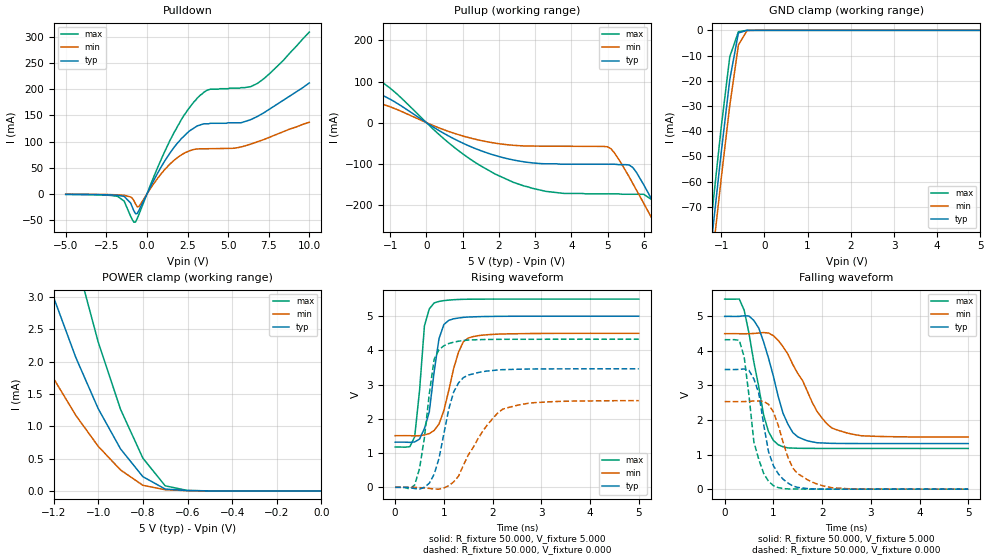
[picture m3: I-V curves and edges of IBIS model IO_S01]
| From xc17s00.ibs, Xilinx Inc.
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|   Model IO_S01
[Model]   IO_S01
Model_type   I/O
Polarity   Non-Inverting
Enable   Active-High
Vinl =   0.800V
Vinh =   2.000V
Vmeas =   2.500V
Cref =  50.000pF
Rref =   1.000M
Vref =  0.000V
C_comp   2.750pF   2.250pF   3.250pF
[Temperature Range]   50.000   100.000   0.000
[Voltage Range]   5.000V   4.500V   5.500V
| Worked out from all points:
|   slope of the pulldown table from 0 to 0.75 V, typ, clamps not added: 16.8 ohm
|   slope of the pullup table from 0 to 0.75 V, typ, clamps not added: 19.3 ohm
|   GND clamp passes 1 mA (typ) near -0.59 V on its own axis
|   POWER clamp passes 1 mA (typ) near -0.96 V on its own axis
|   rising waveform, R_fixture 50.000, V_fixture 5.000: 20-80 % time 222ps typ, 325ps min, 154ps max; typ from 1.32 V to 5 V
|   rising waveform, R_fixture 50.000, V_fixture 0.000: 20-80 % time 331ps typ, 657ps min, 237ps max; typ from 0 V to 3.46 V
|   falling waveform, R_fixture 50.000, V_fixture 5.000: 20-80 % time 444ps typ, 672ps min, 339ps max; typ from 5 V to 1.32 V
|   falling waveform, R_fixture 50.000, V_fixture 0.000: 20-80 % time 296ps typ, 409ps min, 267ps max; typ from 3.46 V to 0 V
[Pulldown]
| voltage   I(typ)   I(min)   I(max)
-5V       -500uA     -400uA     -700uA
-1.8V     -2.5mA     -1.6mA     -4.5mA
-1.4V     -4.5mA     -2.4mA     -13.5mA
-1V       -17.19mA   -5.5mA     -42.5mA
-700mV    -37.46mA   -18.93mA   -53.28mA
-500mV    -31.8mA    -24.06mA   -39.58mA
1.4V      77.3mA     56.57mA    101mA
3.1V      130mA      86.12mA    183mA
3.9V      135mA      86.54mA    200mA
5.8V      136mA      89.89mA    203mA
6.8V      148mA      99.73mA    211mA
10V       212mA      137mA      309mA
[Pullup]
| voltage   I(typ)   I(min)   I(max)
-5V       138mA      75.48mA    233mA
-3.8V     136mA      79.24mA    211mA
-2.2V     104mA      68.39mA    154mA
-1V       56.81mA    38.43mA    83.6mA
1V        -49.62mA   -32.24mA   -75.63mA
2.4V      -90.7mA    -55.01mA   -145mA
3.3V      -100mA     -57.13mA   -167mA
5V        -101mA     -58.64mA   -173mA
5.7V      -109mA     -148mA     -174mA
6.4V      -215mA     -261mA     -198mA
6.8V      -281mA     -327mA     -262mA
10V       -833mA     -863mA     -828mA
[GND_clamp]
| voltage   I(typ)   I(min)   I(max)
-5V       -728mA     -719mA     -739mA
-1.4V     -113mA     -121mA     -104mA
-1.2V     -80.19mA   -89.89mA   -70.7mA
-1V       -48.75mA   -59.03mA   -38.71mA
-800mV    -19.55mA   -29.76mA   -10.47mA
-600mV    -1.037mA   -5.805mA   -545uA
-400mV    -3.699uA   -72.4uA    -2.038uA
5V        350pA      999nA      143pA
[POWER_clamp]
| voltage   I(typ)   I(min)   I(max)
-5V       71.66mA    42.52mA    116mA
-1.4V     5.246mA    3.126mA    8.7mA
-1.3V     4.067mA    2.398mA    6.818mA
-1.2V     3.001mA    1.742mA    5.11mA
-1.1V     2.064mA    1.169mA    3.598mA
-1V       1.274mA    691uA      2.306mA
-900mV    651uA      325uA      1.264mA
-800mV    221uA      87.03uA    508uA
-700mV    28.94uA    18.03uA    79.19uA
-600mV    5.041uA    4.416uA    6.917uA
0V        350pA      2.497nA    186pA
[Ramp]
| variable   typ   min   max
dV/dt_r   2.077/0.321n   1.520/0.637n   2.596/0.184n
dV/dt_f   2.209/0.440n   1.795/0.668n   2.593/0.308n
R_load = 50.000
[Rising Waveform]
R_fixture = 50.000
V_fixture = 5.000
V_fixture_min = 4.500
V_fixture_max = 5.500
L_fixture = 0.000H
C_fixture = 0.000F
| time   V(typ)   V(min)   V(max)
0s        1.319V     1.509V     1.178V
400ps     1.326V     1.504V     1.474V
600ps     1.716V     1.53V      4.712V
700ps     2.203V     1.569V     5.214V
800ps     3.381V     1.66V      5.387V
900ps     4.347V     1.851V     5.431V
1ns       4.757V     2.245V     5.455V
1.3ns     4.947V     3.95V      5.488V
1.5ns     4.975V     4.362V     5.495V
5ns       5V         4.499V     5.5V
[Rising Waveform]
R_fixture = 50.000
V_fixture = 0.000
V_fixture_min = 0.000
V_fixture_max = 0.000
L_fixture = 0.000H
C_fixture = 0.000F
| time   V(typ)   V(min)   V(max)
0s        0V         0V         0V
400ps     -36.91mV   -1.493mV   68.88mV
600ps     2.791mV    -20.69mV   1.452V
800ps     381mV      -52.4mV    3.743V
1ns       1.57V      -19.69mV   4.136V
1.2ns     2.782V     158mV      4.242V
1.3ns     3.05V      324mV      4.268V
1.8ns     3.38V      1.644V     4.317V
2.2ns     3.437V     2.277V     4.324V
5ns       3.462V     2.533V     4.326V
[Falling Waveform]
R_fixture = 50.000
V_fixture = 5.000
V_fixture_min = 4.500
V_fixture_max = 5.500
L_fixture = 0.000H
C_fixture = 0.000F
| time   V(typ)   V(min)   V(max)
0s        5V         4.5V       5.5V
300ps     5V         4.498V     5.501V
400ps     5.017V     4.497V     5.182V
600ps     4.881V     4.506V     3.67V
800ps     4.259V     4.532V     2.14V
1.1ns     2.678V     4.303V     1.284V
1.4ns     1.636V     3.604V     1.189V
1.9ns     1.343V     2.242V     1.179V
2.2ns     1.326V     1.77V      1.179V
5ns       1.319V     1.509V     1.178V
[Falling Waveform]
R_fixture = 50.000
V_fixture = 0.000
V_fixture_min = 0.000
V_fixture_max = 0.000
L_fixture = 0.000H
C_fixture = 0.000F
| time   V(typ)   V(min)   V(max)
0s        3.462V     2.534V     4.326V
300ps     3.466V     2.533V     4.308V
400ps     3.478V     2.535V     3.832V
600ps     3.19V      2.551V     1.364V
700ps     2.777V     2.552V     865mV
800ps     1.875V     2.538V     458mV
1ns       681mV      2.234V     103mV
1.4ns     92.11mV    608mV      4.998mV
1.8ns     7.997mV    202mV      1.287mV
5ns       186uV      382uV      121uV
